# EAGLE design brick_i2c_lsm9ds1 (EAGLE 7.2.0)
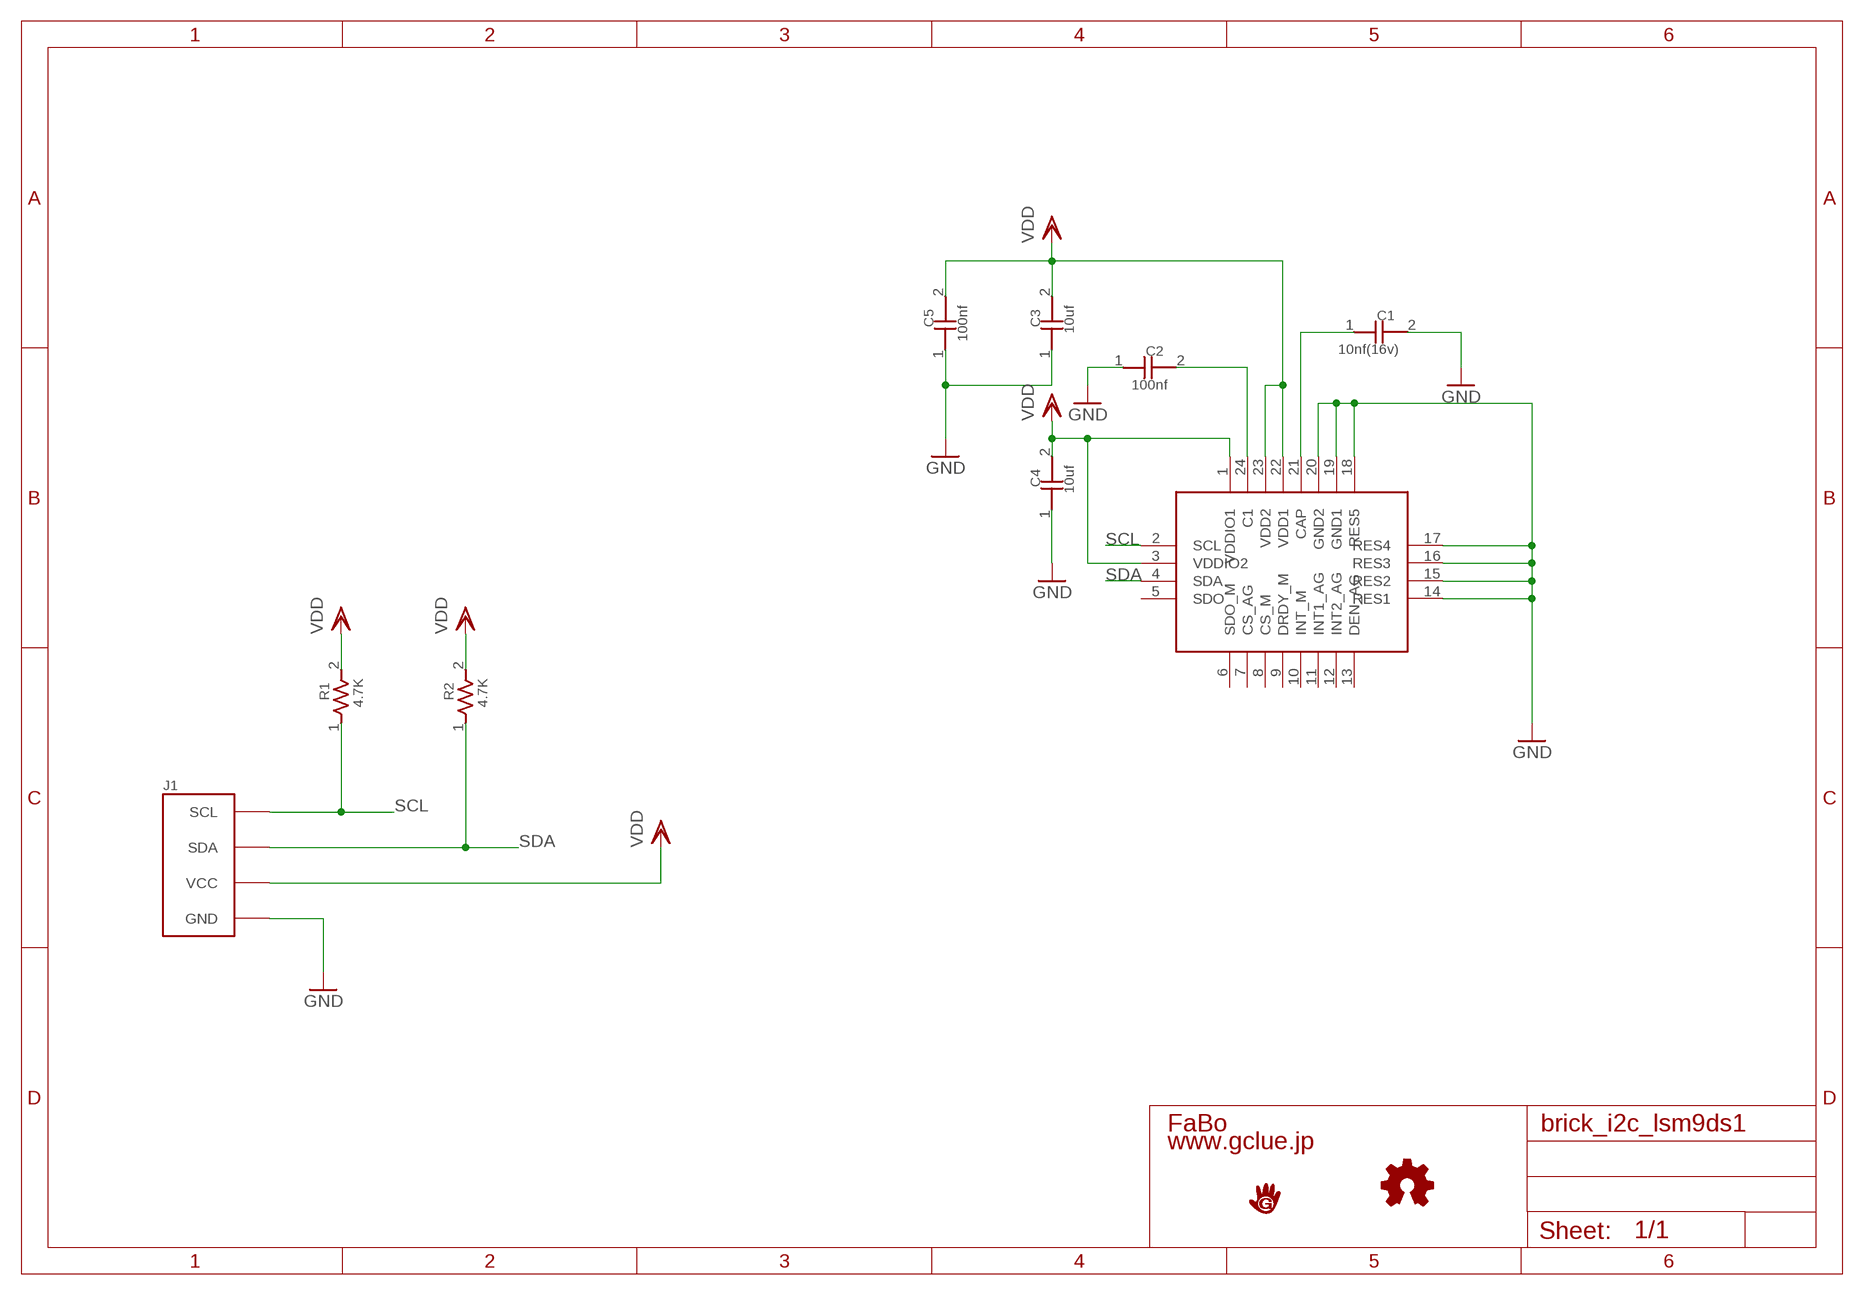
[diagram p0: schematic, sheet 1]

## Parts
C1  10nf(16v)  CAPACITOR0603  [0603]
C2  100nf  CAPACITOR0603  [0603]
C3  10uf  CAPACITOR0603  [0603]
C4  10uf  CAPACITOR0603  [0603]
C5  100nf  CAPACITOR0603  [0603]
J1  BRICK_I2C  [BRICK_I2C]
R1  4.7K  RESISTOR0603  [0603]
R2  4.7K  RESISTOR0603  [0603]
U$1  ST-LSM9DS1TR  [ST-LSM9DS1TR]
U$3  LOGO_GCLUE-M  [LOGO_GCLUE_M]
U$4  LOGO_OSHW-M  [LOGO_OSHW_M]

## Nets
GND: C1.2 C2.1 C3.1 C4.1 C5.1 J1.GND U$1.14(RES1) U$1.15(RES2) U$1.16(RES3) U$1.17(RES4) U$1.18(RES5) U$1.19(GND1) U$1.20(GND2)
N$1: C1.1 U$1.21(CAP)
N$6: C2.2 U$1.24(C1)
SCL: J1.SCL R1.1 U$1.2(SCL)
SDA: J1.SDA R2.1 U$1.4(SDA)
VDD: C3.2 C4.2 C5.2 J1.VCC R1.2 R2.2 U$1.1(VDDIO1) U$1.3(VDDIO2) U$1.22(VDD1) U$1.23(VDD2)
Unconnected: U$1.5(SDO) U$1.6(SDO_M) U$1.7(CS_AG) U$1.8(CS_M) U$1.9(DRDY_M) U$1.10(INT_M) U$1.11(INT1_AG) U$1.12(INT2_AG) U$1.13(DEN_AG)

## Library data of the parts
C1-C5 = GClue-Capacitor:CAPACITOR
J1 = gclue:BRICK_I2C: FaBo Brick 4pin(I2C)
R1 R2 = GClue-Resistors:RESISTOR
U$1 = GClue-Mems:ST-LSM9DS1TR
U$3 = gclue:LOGO_GCLUE
U$4 = gclue:LOGO_OSHW

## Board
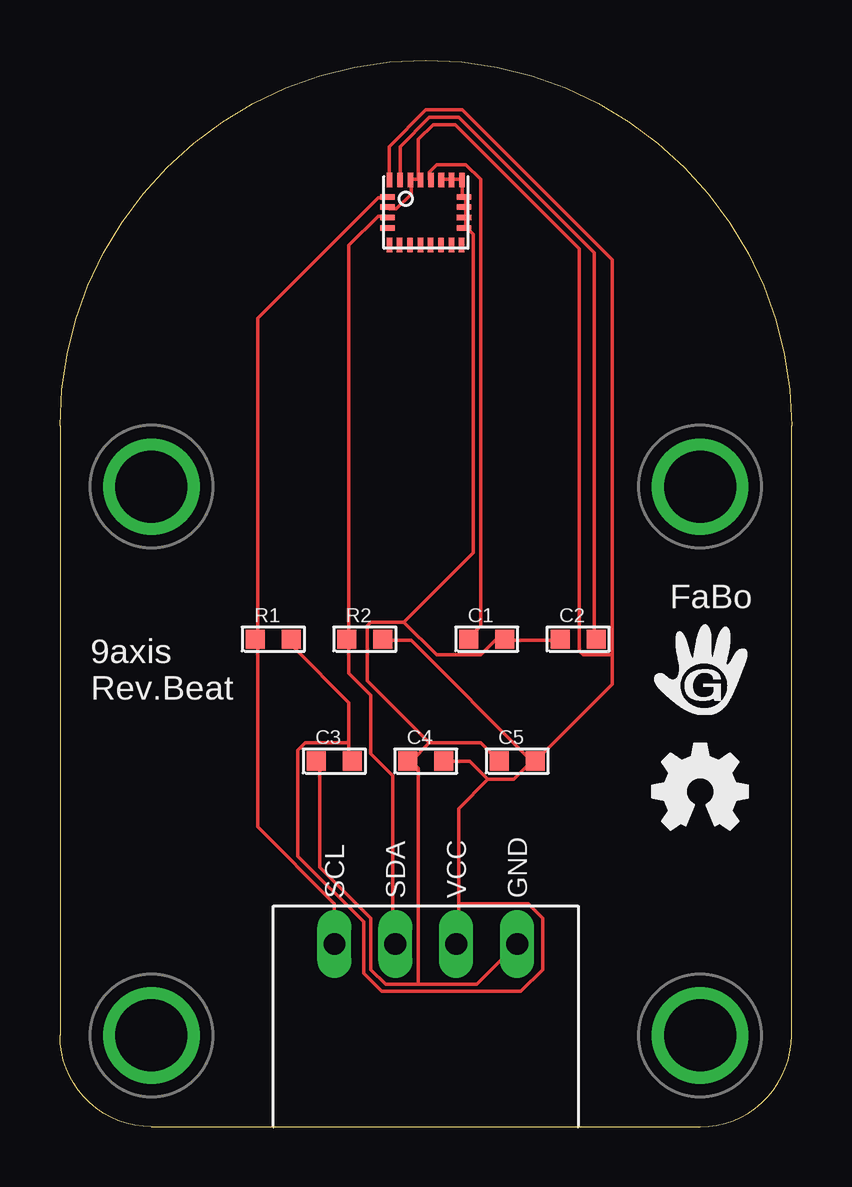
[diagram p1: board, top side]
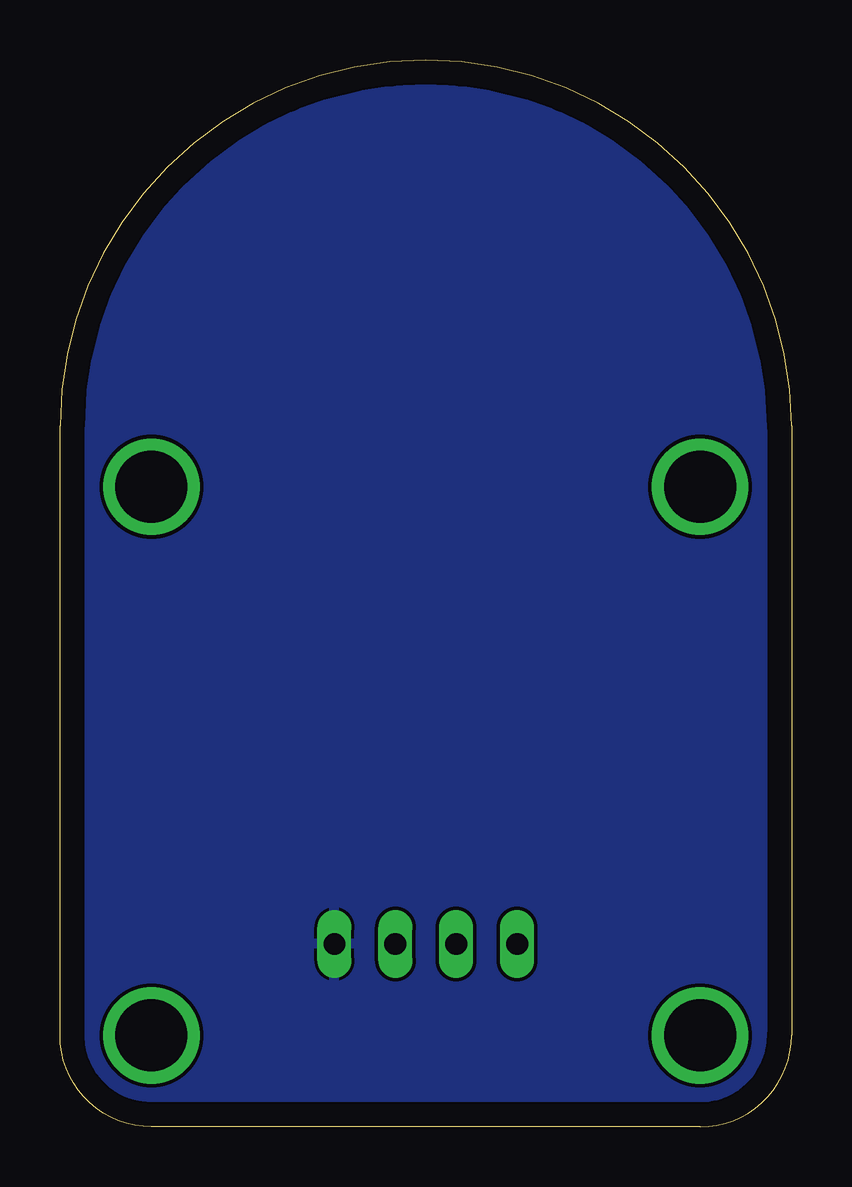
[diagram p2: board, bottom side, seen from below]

Size 30.48 x 44.45 mm. Coordinates in mm from the lower left corner, seen from the top.
Copper layers (1*16): Top 0.035mm / dielectric 1.5mm / Bottom 0.035mm
Design rules "default *": minimum track width 6mil, minimum drill 20mil, track to track 6mil, track to pad 6mil, pad to pad 6mil, via to via 6mil, smd to smd 7mil, copper to edge 40mil, drill to drill 8mil, minimum pad ring 10mil, minimum via ring 8mil, stop-mask expansion 4mil, vias tented up to drill 0mil, thermal gap 5mil

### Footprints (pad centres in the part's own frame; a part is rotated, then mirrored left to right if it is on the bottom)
0603 = smd 0.8 x 0.8: 1 -0.75,0; 2 0.75,0
BRICK_I2C = drill 0.9 long: GND 3.81,-11.43; SCL -3.81,-11.43; SDA -1.27,-11.43; VCC 1.27,-11.43 | drill 3 pad 3.81: P$5 -11.43,7.62; P$6 11.43,7.62; P$7 -11.43,-15.24; P$8 11.43,-15.24
ST-LSM9DS1TR = smd 0.23 x 0.6: 1 -1.505,1.35; 6 -1.517,-1.35; 7 -1.087,-1.35; 8 -0.657,-1.35; 9 -0.227,-1.35; 10 0.203,-1.35; 11 0.633,-1.35; 12 1.063,-1.35; 13 1.493,-1.35; 18 1.505,1.35; 19 1.075,1.35; 20 0.645,1.35; 21 0.215,1.35; 22 -0.215,1.35; 23 -0.645,1.35; 24 -1.075,1.35 | smd 0.6 x 0.23: 2 -1.6,0.648; 3 -1.6,0.218; 4 -1.6,-0.212; 5 -1.6,-0.642; 14 1.6,-0.642; 15 1.6,-0.212; 16 1.6,0.218; 17 1.6,0.648

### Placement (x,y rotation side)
C1  17.78,20.32 0 top
C2  21.59,20.32 0 top
C3  11.43,15.24 0 top
C4  15.24,15.24 0 top
C5  19.05,15.24 0 top
J1  15.24,19.05 0 top
R1  8.89,20.32 0 top
R2  12.7,20.32 0 top
U$1  15.24,38.1 0 top
U$3  26.67,19.05 0 top
U$4  26.67,13.97 0 top

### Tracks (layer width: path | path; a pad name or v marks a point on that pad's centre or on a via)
GND
  Top 0.152: 14.94,5.94 17.37,5.94 J1.GND | 14.94,5.94 13.56,5.94 12.95,6.55 12.95,8.69 10.82,10.82 10.82,15.24 C3.1 | 16.31,39.47 15.85,39.47 U$1.20 | 16.31,39.47 16.76,39.47 U$1.18 16.76,39.32 16.76,38.86 U$1.17 16.92,38.71 16.92,38.41 U$1.16 16.92,38.25 16.92,37.95 U$1.15 16.92,37.8 16.92,37.49 | 16.31,39.47 U$1.19 | C2.1 20.73,20.27 18.59,20.27 C1.2 18.44,20.27 18.14,20.27 17.53,19.66 15.7,19.66 14.33,21.03 | 15.39,16 14.63,15.24 | 15.39,16 17.53,16 18.29,15.24 C5.1 | 14.33,21.03 12.95,21.03 12.8,20.88 12.8,18.59 15.39,16 | 16.92,37.49 17.22,37.19 17.22,23.93 14.33,21.03 | 16.92,37.49 U$1.14 | 14.94,5.94 14.94,14.94 14.63,15.24 | 14.63,15.24 C4.1
  pour Bottom: 0,0 30.48,0 30.48,44.45 0,44.45
N$1
  Top 0.152: U$1.21 15.39,39.47 15.39,39.78 15.7,40.08 16.92,40.08 17.53,39.47 17.53,20.88 17.07,20.42 C1.1
N$6
  Top 0.152: U$1.24 14.17,39.47 14.17,40.84 15.39,42.06 16.61,42.06 22.25,36.42 22.25,20.42 C2.2
SCL
  Top 0.152: U$1.2 13.56,38.71 13.26,38.71 8.23,33.68 8.23,20.42 R1.1 8.23,20.27 8.23,12.5 11.43,9.3 J1.SCL
SDA
  Top 0.152: U$1.4 13.56,37.95 13.26,37.95 12.04,36.73 12.04,20.42 R2.1 12.04,20.27 12.04,18.9 12.95,17.98 12.95,15.54 13.87,14.63 13.87,7.62 J1.SDA
VDD
  Top 0.152: 12.04,16 12.04,17.68 9.75,19.96 9.75,20.27 R1.2 | 12.04,16 12.04,15.24 C3.2 | U$1.3 13.72,38.25 14.02,38.25 14.63,38.86 14.63,39.32 U$1.23 14.63,39.47 14.94,39.47 | 23.01,19.66 23.01,18.44 19.81,15.24 C5.2 19.66,15.24 | 23.01,19.66 23.01,36.12 16.76,42.37 15.24,42.37 13.72,40.84 13.72,39.47 U$1.1 | C4.2 17.07,15.24 17.83,14.48 | 17.83,14.48 18.9,14.48 19.66,15.24 | 19.66,15.24 14.63,20.27 13.56,20.27 R2.2 | 14.94,39.47 14.94,41.15 15.54,41.76 16.46,41.76 21.64,36.58 21.64,19.81 21.79,19.66 23.01,19.66 | 14.94,39.47 U$1.22 | 16.61,9.3 16.61,13.26 17.83,14.48 | 16.61,9.3 16.61,7.62 J1.VCC | 12.04,16 10.21,16 9.91,15.7 9.91,11.28 12.65,8.53 12.65,6.4 13.41,5.64 19.2,5.64 20.12,6.55 20.12,8.69 19.51,9.3 16.61,9.3

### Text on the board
tPlace: FaBo | 9axis / Rev.Beat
